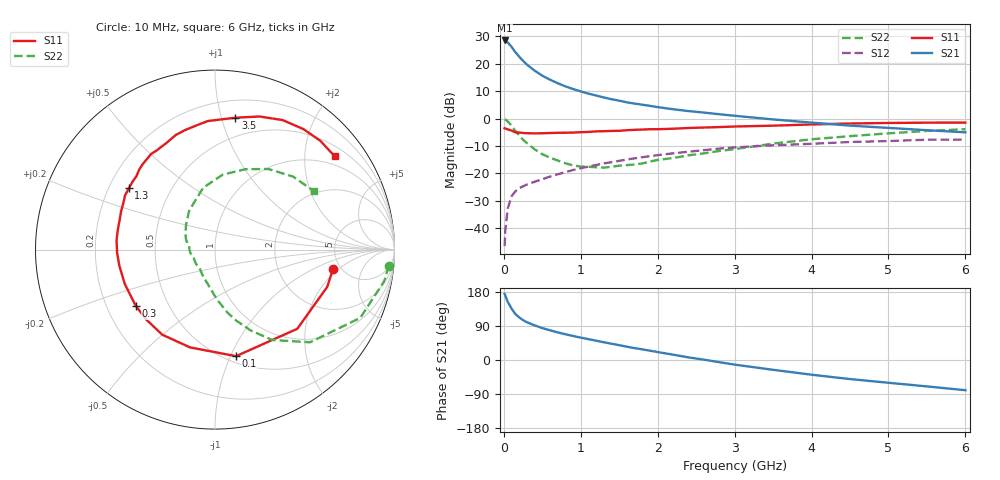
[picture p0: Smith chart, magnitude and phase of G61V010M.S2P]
! SIEMENS Small Signal Semiconductors
! BFG193
! Si NPN RF Bipolar Junction Transistor in SOT223
! VCE = 1 V  IC = 10 mA
! Common Emitter S-Parameters:  August  1996
# GHz  S  MA  R  50
!  f  S11  S21  S12  S22
! GHz  MAG  ANG  MAG  ANG  MAG  ANG  MAG  ANG
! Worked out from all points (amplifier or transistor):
!   36 points, 10 MHz to 6 GHz, reference 50 ohm
!   highest |S21| = 28.5 dB at 10 MHz (marker M1)
!   |S21| within 3 dB of that: start of sweep to 117 MHz
!   unconditionally stable (mu >= 1): 817.4 MHz to 2.979 GHz
!   at 250 MHz: K = 0.55, MSG = 22.9 dB, |S12| = -24.7 dB
!   at 1.4 GHz: K = 1.08, MAG = 9.7 dB, |S12| = -15.9 dB
!   at 6 GHz: K = 0.96, MSG = 1.3 dB, |S12| = -7.7 dB
!   S11 on the Smith chart (normalised r, x): 10 MHz: 4.32, -1.68; 100 MHz: 0.56, -1.05; 300 MHz: 0.32, -0.29; 1.3 GHz: 0.28, +0.30; 3.5 GHz: 0.34, +1.11; 6 GHz: 0.75, +2.72
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0.01  0.6667 -9.3  26.69 174.4  0.0047 89.5  0.9722 -5.3
0.02  0.6587 -18.4  26.54 169.7  0.0094 83.0  0.959 -10.6
0.05  0.6363 -43.9  24.67 153.8  0.0227 70.6  0.8942 -25.2
0.1  0.6052 -78.8  20.39 135.6  0.0383 58.5  0.7394 -44.3
0.15  0.5624 -104.3  16.3 121.3  0.0471 50.8  0.5957 -57.7
0.2  0.5578 -121.8  13.49 112.4  0.0537 47.2  0.4923 -66.2
0.25  0.5464 -134.7  11.29 105.1  0.0581 45.1  0.4111 -73.5
0.3  0.5412 -144.7  9.679 99.6  0.0627 44.8  0.3568 -78.9
0.4  0.5379 -159.2  7.505 91.4  0.0705 44.8  0.2752 -88.1
0.5  0.5404 -170.4  6.072 84.2  0.0785 45.1  0.224 -95.6
0.6  0.5458 -178.2  5.13 78.4  0.0875 45.6  0.1939 -102.4
0.7  0.5507 174.6  4.429 72.8  0.0963 45.9  0.1718 -110.3
0.8  0.5526 168.9  3.878 68.0  0.1054 45.3  0.1534 -118.4
1.1  0.5718 153.4  2.859 55.0  0.1333 43.6  0.1324 -142.1
1.3  0.5893 144.6  2.432 46.8  0.1522 41.3  0.1275 -159.0
1.7  0.6241 130.1  1.878 31.3  0.1885 35.1  0.1454 173.3
2.2  0.6531 114.4  1.483 14.1  0.2327 25.0  0.1909 149.2
2.8  0.701 98.0  1.202 -5.7  0.2836 12.2  0.2568 124.6
3.5  0.7436 81.2  0.966 -25.9  0.326 -4.5  0.3501 101.0
4.5  0.8142 62.4  0.745 -50.3  0.3744 -23.6  0.4788 69.3
5.5  0.8437 45.9  0.614 -69.7  0.4123 -46.1  0.5954 43.1
6  0.8455 38.0  0.562 -79.7  0.4135 -59.1  0.6407 30.5
